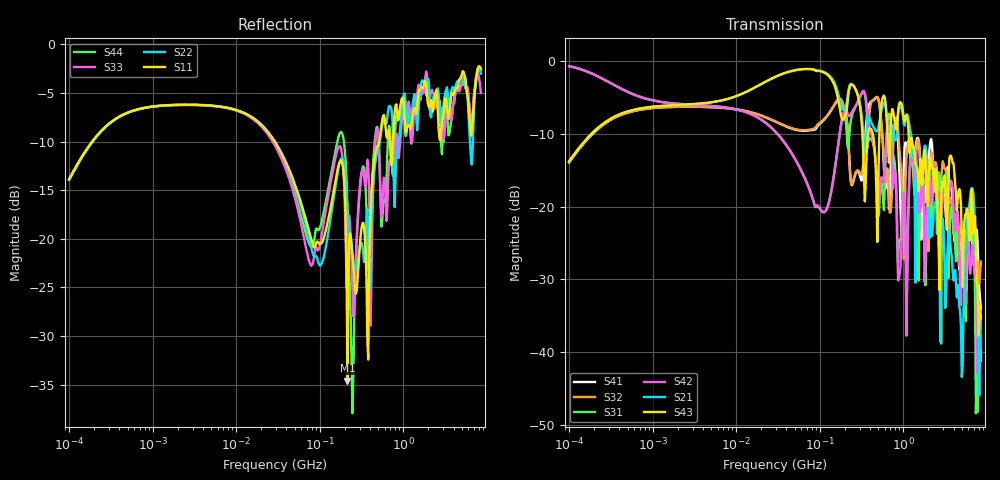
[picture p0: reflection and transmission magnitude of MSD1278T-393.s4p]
# MHz S MA R 50
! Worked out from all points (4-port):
!   498 points, 100 kHz to 8.5 GHz, reference 50 ohm
!   strongest paths, dB at 100 kHz, 1.698 MHz, 29.49 MHz, 500.7 MHz, 8.5 GHz:
!     S43: -13.7, -6.1, -2.1, -17.9, -35.3
!     S21: -13.8, -6.1, -2.2, -9.3, -35.0
!     S42: -0.7, -5.8, -9.7, -20.0, -35.6
!     S31: -0.7, -5.8, -9.7, -21.4, -41.2
!     S32: -13.9, -6.3, -8.3, -5.1, -27.6
!     S41: -13.9, -6.3, -8.3, -5.1, -34.0
!   lowest |S11| = -34.6 dB at 215.1 MHz (marker M1), VSWR 1.04, Z = 51 + j1.57 ohm
!   |S11| at or under -10 dB: start of sweep to 189.3 kHz; 29.1 MHz to 514.9 MHz (485.8 MHz wide, 179 % of centre); 692.2 MHz to 753.5 MHz (61.29 MHz wide, 8.48 % of centre)
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0.1  0.2028 63.7  0.205 64.6  0.9241 -11.6  0.2013 -116.0
     0.205 64.6  0.2002 64.0  0.2013 -115.9  0.9247 -11.6
     0.9241 -11.6  0.2013 -115.9  0.202 64.0  0.2054 64.4
     0.2013 -116.0  0.9247 -11.6  0.2054 64.4  0.2022 64.4
215.0626  0.01865 55.6  0.5661 -33.3  0.259 33.9  0.3609 -52.9
          0.5661 -33.3  0.1353 -118.7  0.3495 -58.3  0.4366 43.7
          0.259 33.9  0.3495 -58.3  0.08627 52.6  0.5124 -31.6
          0.3609 -52.9  0.4366 43.7  0.5124 -31.6  0.1463 -122.5
246.6465  0.08387 -113.8  0.6919 -55.4  0.4353 33.6  0.1418 -26.3
          0.6919 -55.4  0.0807 -156.0  0.1451 -27.5  0.4546 26.4
          0.4353 33.6  0.1451 -27.5  0.05359 -37.0  0.6879 -57.7
          0.1418 -26.3  0.4546 26.4  0.6879 -57.7  0.01267 162.3
3111.8  0.4905 83.4  0.04238 -39.0  0.1514 35.8  0.1281 24.3
        0.04238 -39.0  0.5299 79.9  0.1836 35.3  0.1356 43.0
        0.1514 35.8  0.1836 35.3  0.3389 74.6  0.1631 26.7
        0.1281 24.3  0.1356 43.0  0.1631 26.7  0.405 91.2
5026.862  0.7028 -89.6  0.006738 72.8  0.05015 -147.0  0.05305 -159.8
          0.006738 72.8  0.6616 -102.3  0.05546 -152.4  0.03852 -130.4
          0.05015 -147.0  0.05546 -152.4  0.6495 -97.4  0.05983 89.1
          0.05305 -159.8  0.03852 -130.4  0.05983 89.1  0.6196 -91.2
6611.76  0.3518 95.5  0.1344 30.9  0.08298 30.2  0.06227 61.3
         0.1344 30.9  0.2409 115.6  0.1101 38.3  0.05412 66.8
         0.08298 30.2  0.1101 38.3  0.3344 96.7  0.1318 10.0
         0.06227 61.3  0.05412 66.8  0.1318 10.0  0.3831 136.3
8500  0.7521 -55.4  0.01774 -42.0  0.008694 -117.8  0.01997 -162.3
      0.01774 -42.0  0.7071 -64.3  0.04189 164.9  0.01663 -82.0
      0.008694 -117.8  0.04189 164.9  0.5626 -62.0  0.0171 -76.9
      0.01997 -162.3  0.01663 -82.0  0.0171 -76.9  0.7415 -56.0
